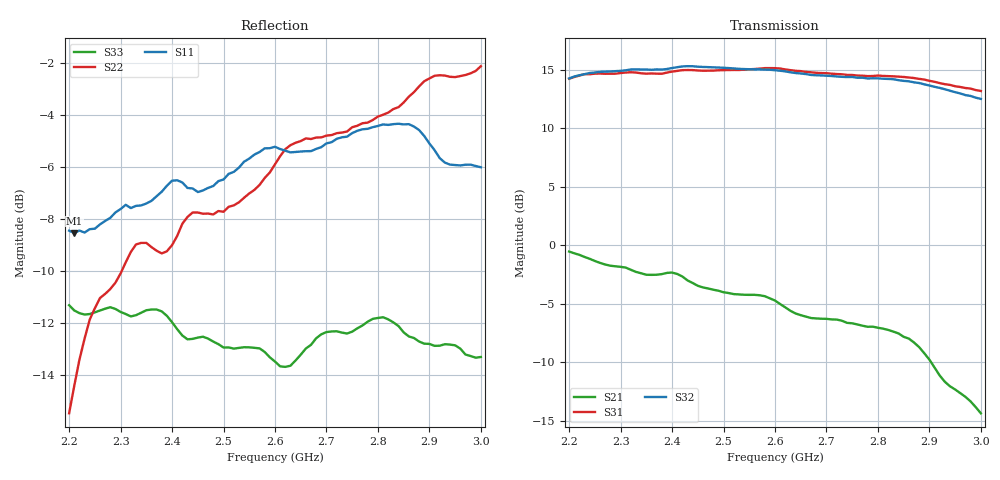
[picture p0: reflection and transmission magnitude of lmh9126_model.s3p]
! Created Sun Feb 16 19:39:56 2020
# hz S ri R 50
! 3 Port Network Data from SP1.SP block
! freq  reS11  imS11  reS12  imS12  reS13  imS13
!  reS21  imS21
!  reS22  imS22  reS23  imS23
!  reS31  imS31  reS32  imS32
!  reS33  imS33
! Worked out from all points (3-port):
!   81 points, 2.2 GHz to 3 GHz, reference 50 ohm
!   strongest paths, dB at 2.2 GHz, 2.4 GHz, 2.6 GHz, 2.8 GHz, 3 GHz:
!     S32: 14.2, 15.1, 15.0, 14.3, 12.5
!     S31: 14.2, 14.8, 15.1, 14.5, 13.2
!     S21: -0.5, -2.3, -4.7, -7.0, -14.3
!   lowest |S11| = -8.5 dB at 2.21 GHz (marker M1), VSWR 2.20, Z = 36.8 - j32 ohm
!   |S11| at or under -10 dB: nowhere
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2.2e9  -0.00614 -0.3782  0.0904 -0.4634  -0.0427 -0.00166
       -0.1183 -0.9326  0.1674 -0.0213  -0.0453 -0.0256
       0.4103 5.124  -0.5477 -5.128  0.0136 -0.2717
2.21e9  -0.0148 -0.3741  0.0923 -0.4576  -0.042 -0.000649
        -0.1434 -0.913  0.1885 -0.0273  -0.0465 -0.0229
        0.646 5.191  -0.77 -5.197  0.00803 -0.2657
2.32e9  -0.0513 -0.4148  0.1058 -0.4124  -0.0369 0.00508
        -0.2597 -0.7416  0.2967 -0.1748  -0.0388 -0.0135
        2.886 4.658  -3.005 -4.763  -0.0954 -0.2407
2.44e9  -0.1693 -0.4232  0.1432 -0.3924  -0.0347 0.00641
        -0.3585 -0.59  0.2734 -0.3054  -0.0405 -0.0135
        4.509 3.314  -4.798 -3.282  -0.1875 -0.1407
2.51e9  -0.2318 -0.4273  0.1357 -0.3762  -0.0289 0.00561
        -0.3533 -0.5157  0.1706 -0.3841  -0.0347 -0.015
        5.12 2.262  -5.326 -2.053  -0.2154 -0.0676
2.6e9  -0.3523 -0.4198  0.1812 -0.3572  -0.0309 -0.00295
       -0.4158 -0.4055  0.1432 -0.4866  -0.043 -0.0248
       5.665 0.6766  -5.57 -0.4854  -0.2019 0.0648
2.75e9  -0.4607 -0.3559  0.2185 -0.3911  -0.0328 -0.0106
        -0.393 -0.2474  0.0638 -0.594  -0.0502 -0.0279
        5.034 -1.762  -4.929 1.752  -0.1393 0.198
2.86e9  -0.5658 -0.2162  0.235 -0.4771  -0.0538 -0.0191
        -0.3955 -0.0567  -0.0654 -0.6807  -0.0778 -0.0295
        4.056 -3.259  -3.882 3.171  0.00508 0.2369
2.93e9  -0.4982 -0.1135  0.1591 -0.5273  -0.0628 -0.00267
        -0.259 0.0347  -0.2294 -0.7148  -0.0859 -0.00699
        3.05 -3.799  -2.881 3.631  0.0531 0.2227
3e9  -0.4988 -0.0423  0.1018 -0.5285  -0.0668 0.00632
     -0.1792 0.0682  -0.3645 -0.6925  -0.0856 0.00562
     2.1 -4.045  -1.986 3.718  0.0972 0.1934
